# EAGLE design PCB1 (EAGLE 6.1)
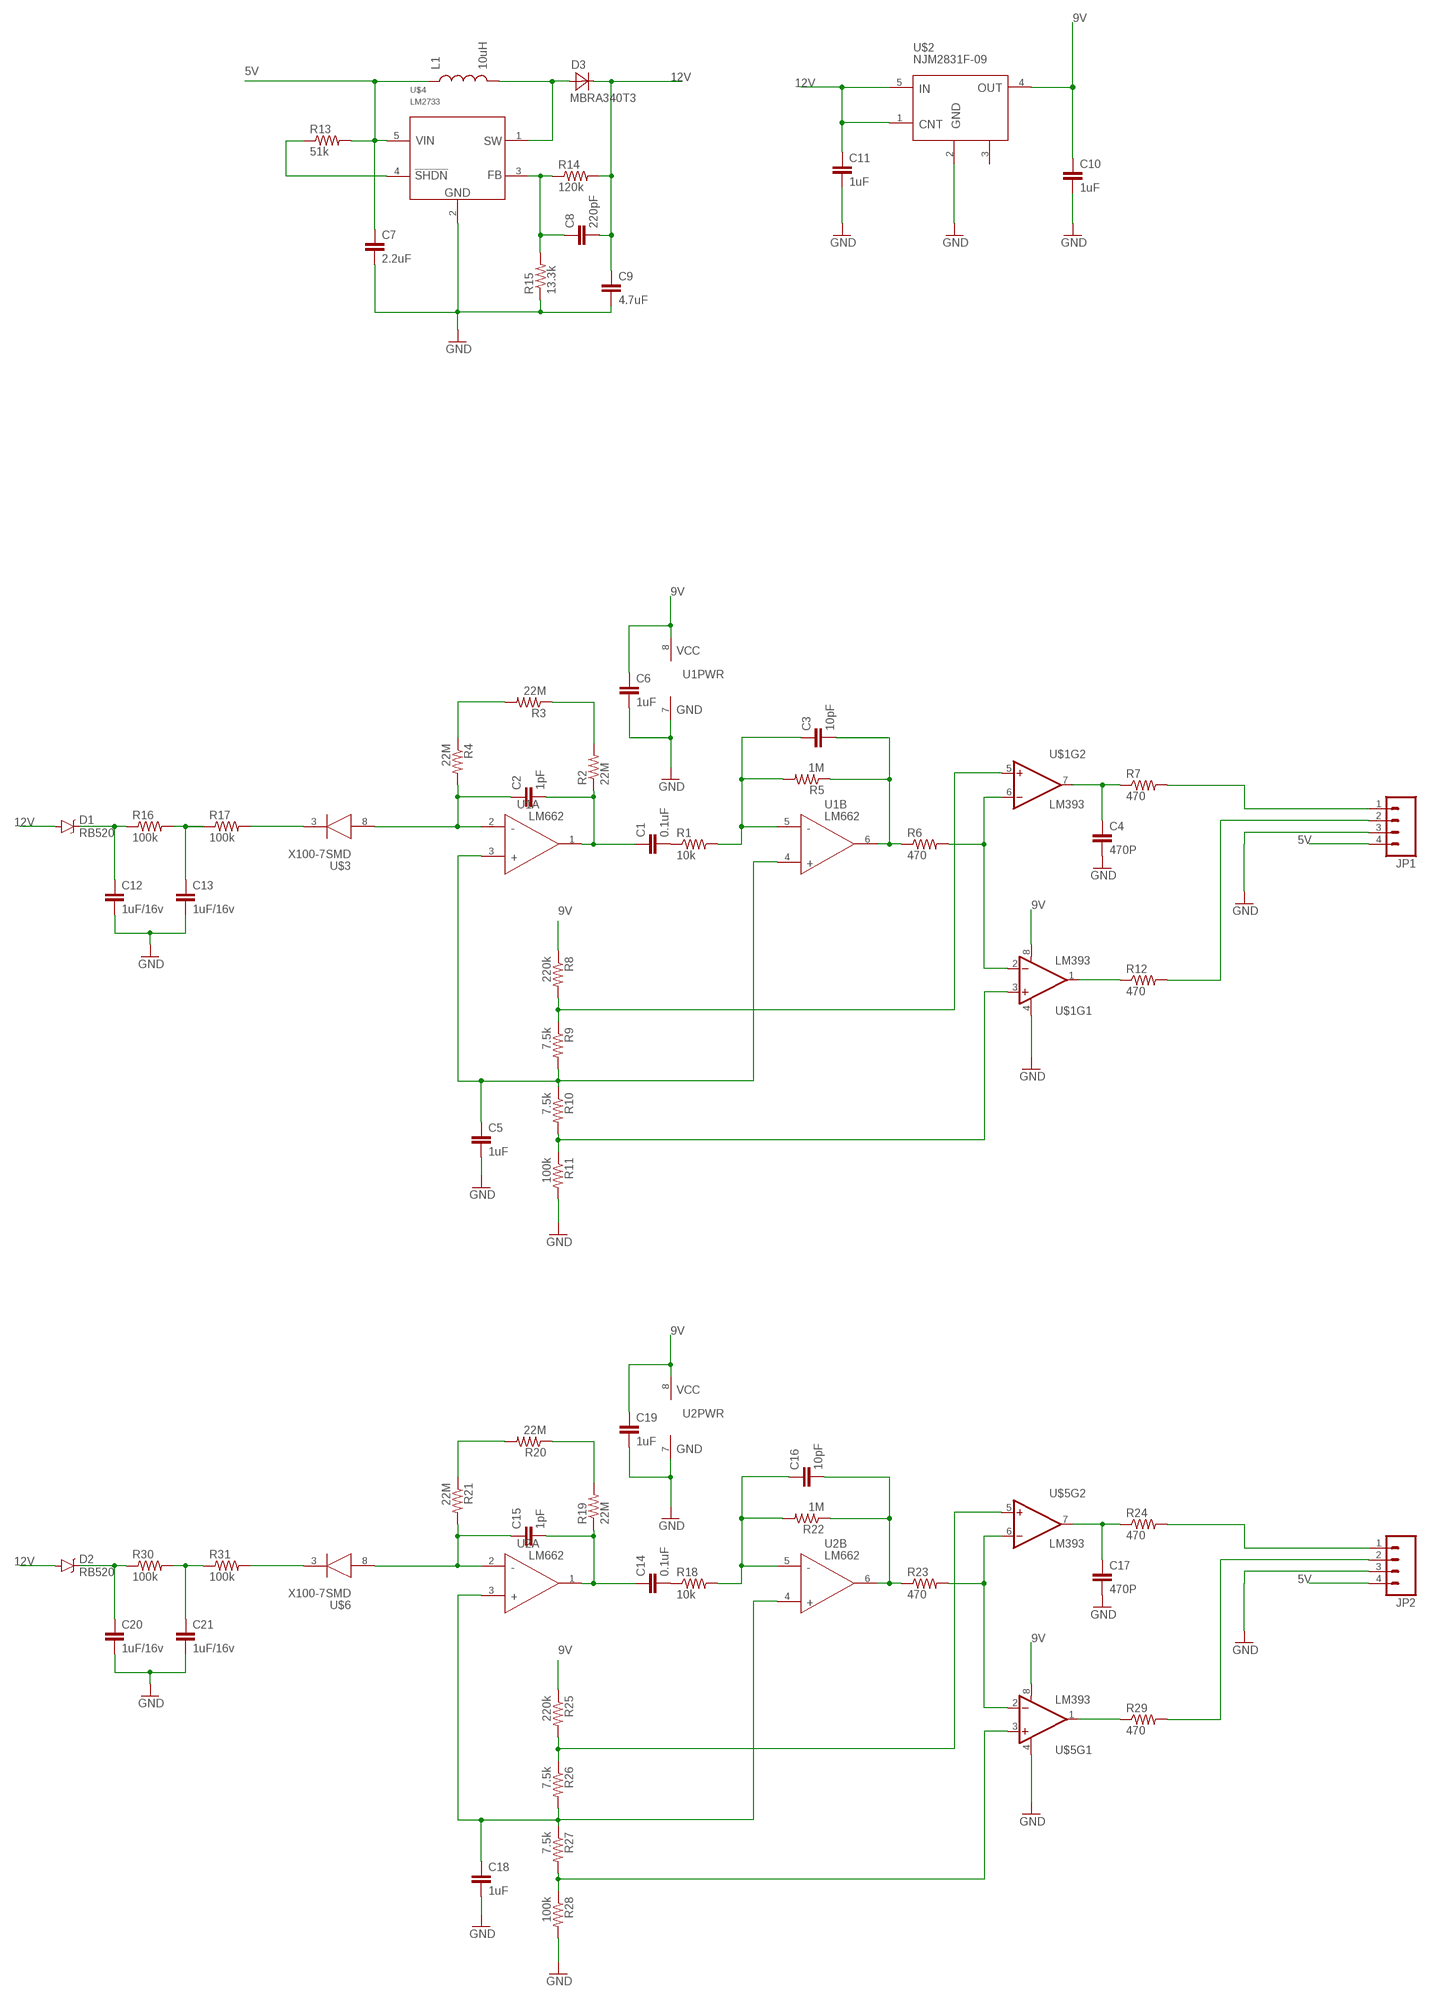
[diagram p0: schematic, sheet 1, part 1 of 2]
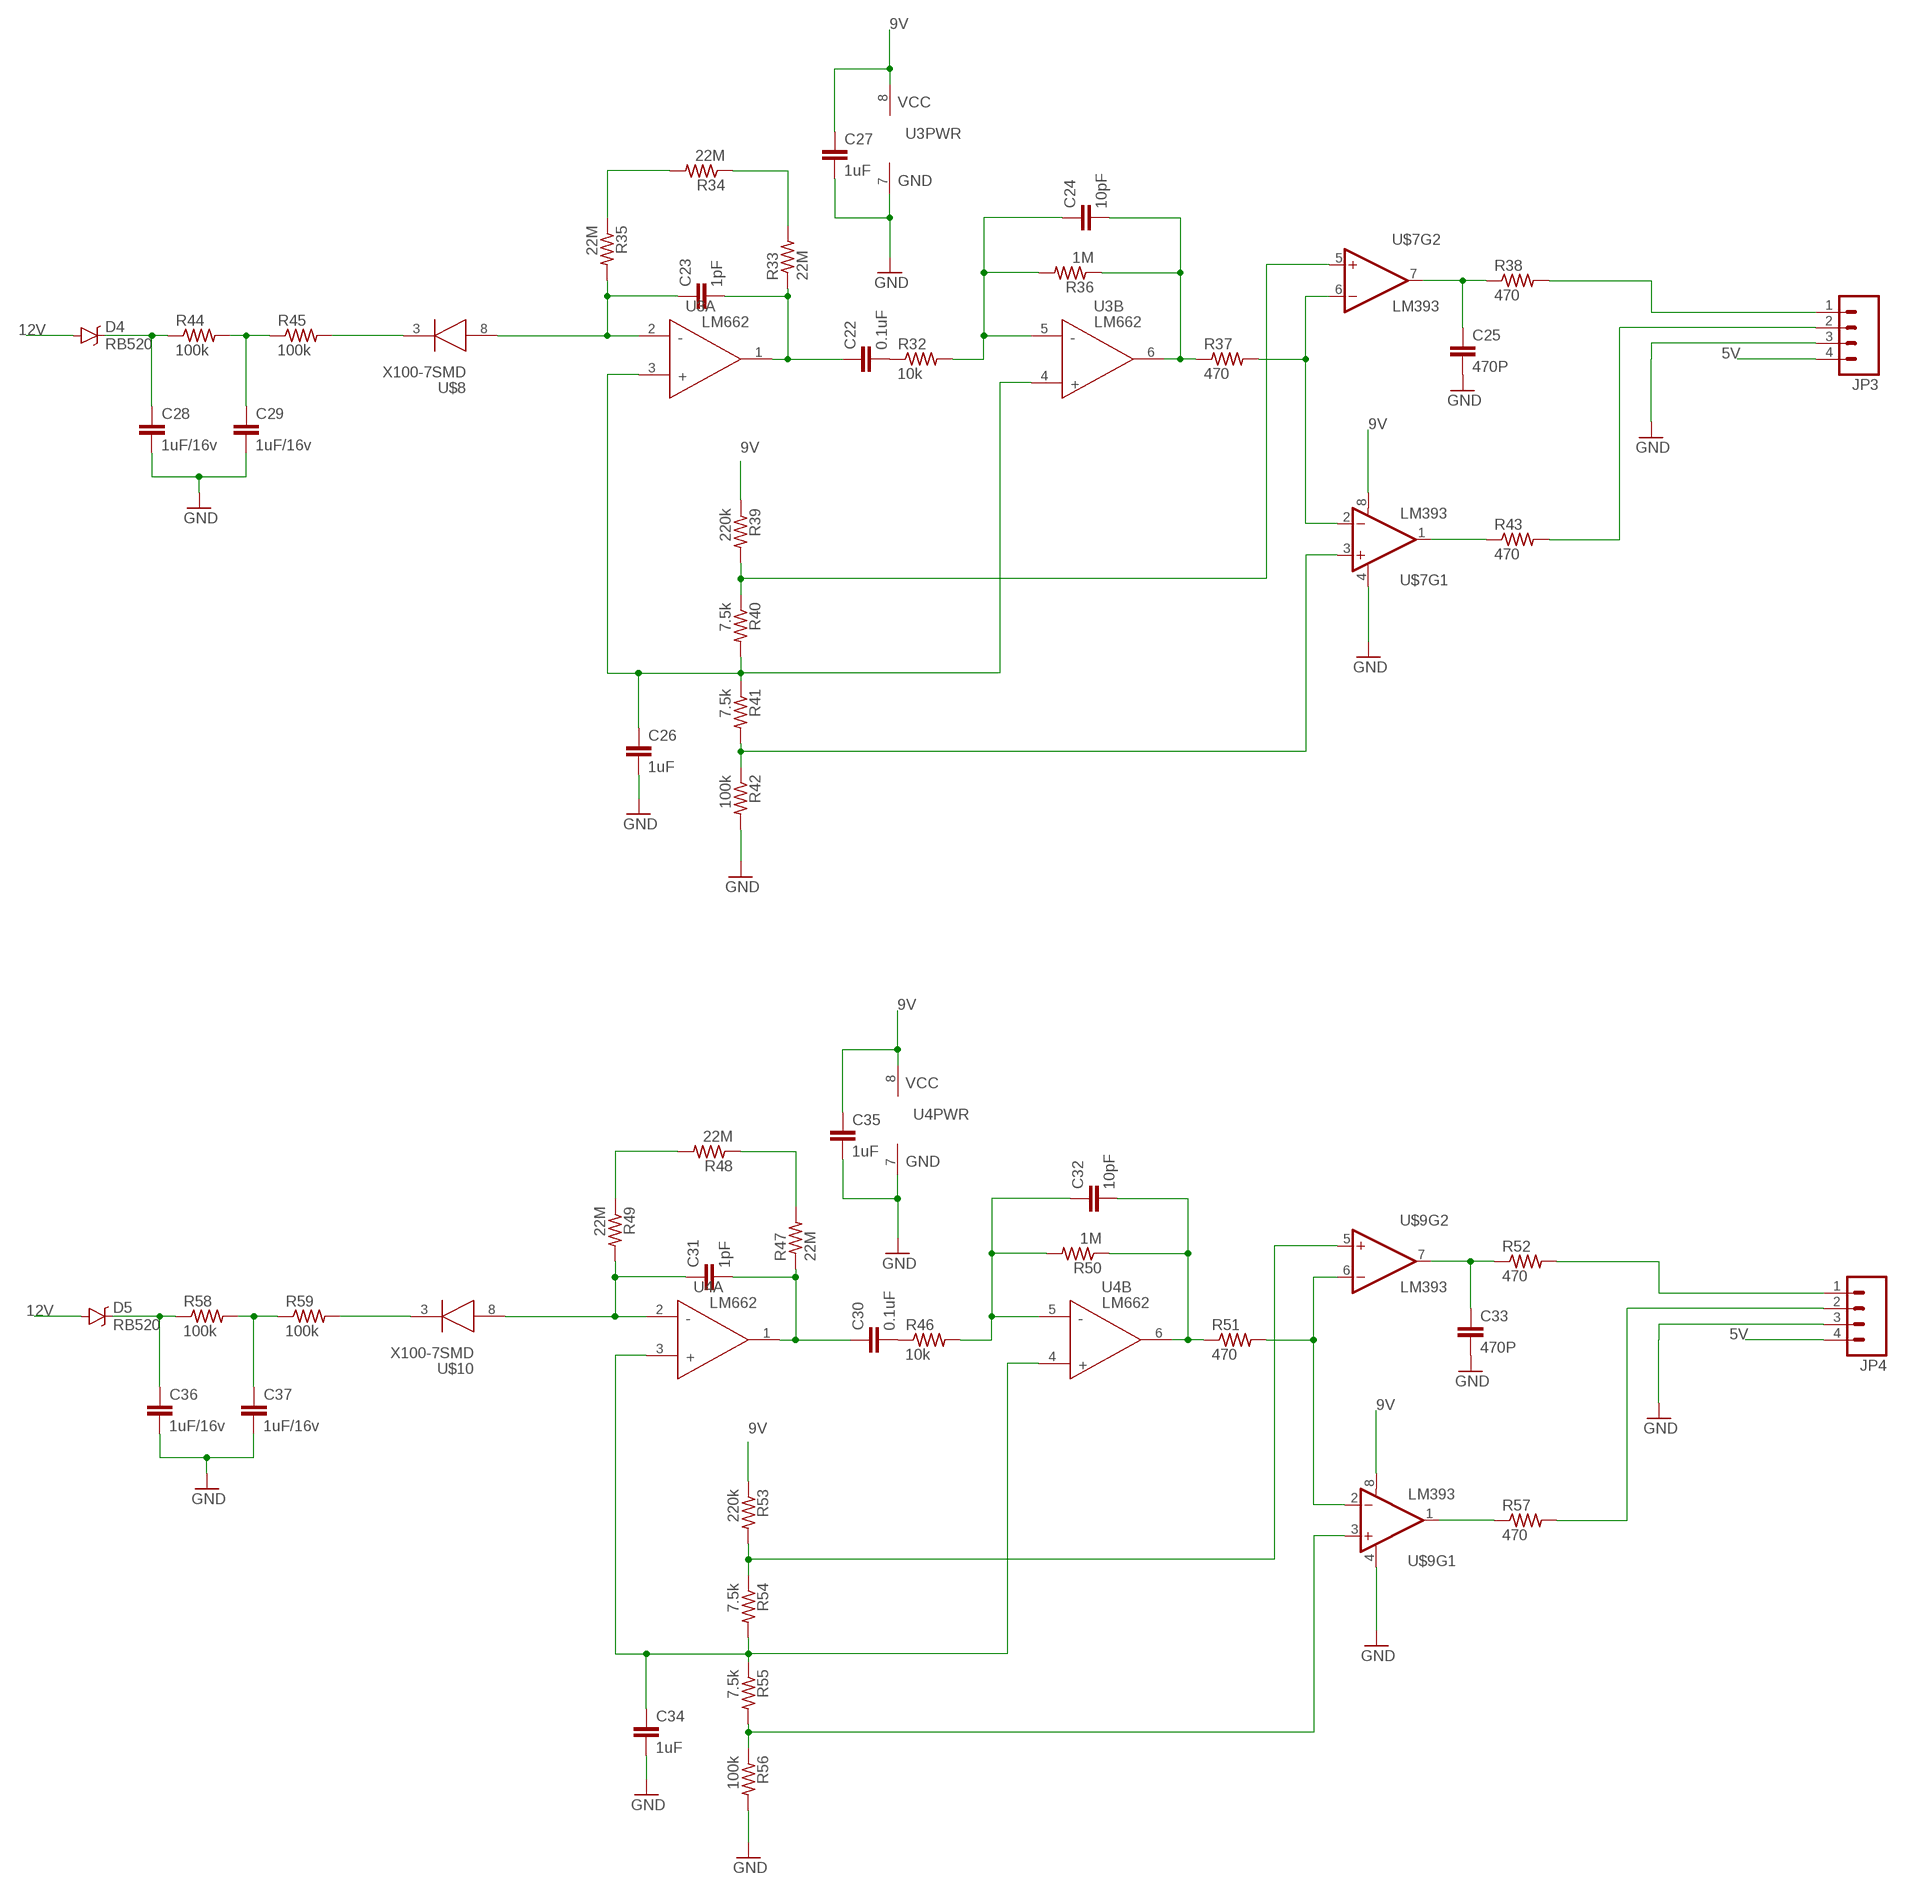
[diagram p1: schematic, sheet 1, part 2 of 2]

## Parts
C1  0.1uF  C-EUC1206  [C1206]
C2  1pF  C-EUC1206  [C1206]
C3  10pF  C-EUC1206  [C1206]
C4  470P  C-EUC1206  [C1206]
C5  1uF  C-EUC1206  [C1206]
C6  1uF  C-EUC1206  [C1206]
C7  2.2uF  C-EUC1206  [C1206]
C8  220pF  C-EUC1206  [C1206]
C9  4.7uF  C-EUC1206  [C1206]
C10  1uF  C-EUC1206  [C1206]
C11  1uF  C-EUC1206  [C1206]
C12  1uF/16v  C-EUC1206  [C1206]
C13  1uF/16v  C-EUC1206  [C1206]
C14  0.1uF  C-EUC1206  [C1206]
C15  1pF  C-EUC1206  [C1206]
C16  10pF  CAP0603-CAP  [0603-CAP]
C17  470P  C-EUC1206  [C1206]
C18  1uF  C-EUC1206  [C1206]
C19  1uF  C-EUC1206  [C1206]
C20  1uF/16v  C-EUC1206  [C1206]
C21  1uF/16v  C-EUC1206  [C1206]
C22  0.1uF  C-EUC1206  [C1206]
C23  1pF  C-EUC1206  [C1206]
C24  10pF  C-EUC1206  [C1206]
C25  470P  C-EUC1206  [C1206]
C26  1uF  C-EUC1206  [C1206]
C27  1uF  C-EUC1206  [C1206]
C28  1uF/16v  C-EUC1206  [C1206]
C29  1uF/16v  C-EUC1206  [C1206]
C30  0.1uF  C-EUC1206  [C1206]
C31  1pF  C-EUC1206  [C1206]
C32  10pF  C-EUC1206  [C1206]
C33  470P  C-EUC1206  [C1206]
C34  1uF  C-EUC1206  [C1206]
C35  1uF  C-EUC1206  [C1206]
C36  1uF/16v  C-EUC1206  [C1206]
C37  1uF/16v  C-EUC1206  [C1206]
D1  RB520  DIODE-SCHOTTKY-RB751  [SOD-523]
D2  RB520  DIODE-SCHOTTKY-RB751  [SOD-523]
D3  MBRA340T3  [SMA]
D4  RB520  DIODE-SCHOTTKY-RB751  [SOD-523]
D5  RB520  DIODE-SCHOTTKY-RB751  [SOD-523]
JP1  M04PTH  [1X04]
JP2  M04PTH  [1X04]
JP3  M04PTH  [1X04]
JP4  M04PTH  [1X04]
L1  10uH  INDUCTORBOURNS_SRN6045  [SRN6045]
R1  10k  R-US_R1206  [R1206]
R2  22M  R-US_R1206  [R1206]
R3  22M  R-US_R1206  [R1206]
R4  22M  R-US_R1206  [R1206]
R5  1M  R-US_R1206  [R1206]
R6  470  R-US_R1206  [R1206]
R7  470  R-US_R1206  [R1206]
R8  220k  R-US_R1206  [R1206]
R9  7.5k  R-US_R1206  [R1206]
R10  7.5k  R-US_R1206  [R1206]
R11  100k  R-US_R1206  [R1206]
R12  470  R-US_R1206  [R1206]
R13  51k  R-US_R1206  [R1206]
R14  120k  R-US_R1206  [R1206]
R15  13.3k  R-US_R1206  [R1206]
R16  100k  R-US_R1206  [R1206]
R17  100k  R-US_R1206  [R1206]
R18  10k  R-US_R1206  [R1206]
R19  22M  R-US_R1206  [R1206]
R20  22M  R-US_R1206  [R1206]
R21  22M  R-US_R1206  [R1206]
R22  1M  R-US_R1206  [R1206]
R23  470  R-US_R1206  [R1206]
R24  470  R-US_R1206  [R1206]
R25  220k  R-US_R1206  [R1206]
R26  7.5k  R-US_R1206  [R1206]
R27  7.5k  R-US_R1206  [R1206]
R28  100k  R-US_R1206  [R1206]
R29  470  R-US_R1206  [R1206]
R30  100k  R-US_R1206  [R1206]
R31  100k  R-US_R1206  [R1206]
R32  10k  R-US_R1206  [R1206]
R33  22M  R-US_R1206  [R1206]
R34  22M  R-US_R1206  [R1206]
R35  22M  R-US_R1206  [R1206]
R36  1M  R-US_R1206  [R1206]
R37  470  R-US_R1206  [R1206]
R38  470  R-US_R1206  [R1206]
R39  220k  R-US_R1206  [R1206]
R40  7.5k  R-US_R1206  [R1206]
R41  7.5k  R-US_R1206  [R1206]
R42  100k  R-US_R1206  [R1206]
R43  470  R-US_R1206  [R1206]
R44  100k  R-US_R1206  [R1206]
R45  100k  R-US_R1206  [R1206]
R46  10k  R-US_R1206  [R1206]
R47  22M  R-US_R1206  [R1206]
R48  22M  R-US_R1206  [R1206]
R49  22M  R-US_R1206  [R1206]
R50  1M  R-US_R1206  [R1206]
R51  470  R-US_R1206  [R1206]
R52  470  R-US_R1206  [R1206]
R53  220k  R-US_R1206  [R1206]
R54  7.5k  R-US_R1206  [R1206]
R55  7.5k  R-US_R1206  [R1206]
R56  100k  R-US_R1206  [R1206]
R57  470  R-US_R1206  [R1206]
R58  100k  R-US_R1206  [R1206]
R59  100k  R-US_R1206  [R1206]
U1  LM662  [SO08]
U2  LM662  [SO08]
U3  LM662  [SO08]
U4  LM662  [SO08]
U$1  LM393  [SO08]
U$2  NJM2831F-09  [SOT23-5]
U$3  X100-7SMD  [X100-7SMD]
U$4  LM2733  [SOT23-5]
U$5  LM393  [SO08]
U$6  X100-7SMD  [X100-7SMD]
U$7  LM393  [SO08]
U$8  X100-7SMD  [X100-7SMD]
U$9  LM393  [SO08]
U$10  X100-7SMD  [X100-7SMD]

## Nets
5V: C7.1 JP1.4 JP2.4 JP3.4 JP4.4 L1.1 R13.2 U$4.5
9V: C6.1 C10.1 C19.1 C27.1 C35.1 R8.1 R25.1 R39.1 R53.1 U1.8 U2.8 U3.8 U4.8 U$1.8(V+) U$2.4 U$5.8(V+) U$7.8(V+) U$9.8(V+)
12V: C8.2 C9.1 C11.1 D1.A D2.A D3.C D4.A D5.A R14.2 U$2.1 U$2.5
GND: C4.2 C5.2 C6.2 C7.2 C9.2 C10.2 C11.2 C12.2 C13.2 C17.2 C18.2 C19.2 C20.2 C21.2 C25.2 C26.2 C27.2 C28.2 C29.2 C33.2 C34.2 C35.2 C36.2 C37.2 JP1.3 JP2.3 JP3.3 JP4.3 R11.2 R15.1 R28.2 R42.2 R56.2 U1.7 U2.7 U3.7 U4.7 U$1.4(V-) U$2.2 U$4.2 U$5.4(V-) U$7.4(V-) U$9.4(V-)
N$1: C1.1 C2.2 R2.1 U1.1
N$2: C1.2 R1.1
N$3: C3.1 R1.2 R5.2 U1.5
N$4: R2.2 R3.1
N$5: R3.2 R4.1
N$6: C2.1 R4.2 U1.2 U$3.8
N$7: C3.2 R5.1 R6.1 U1.6
N$8: R6.2 U$1.2(-IN) U$1.6(-IN)
N$9: C4.1 R7.1 U$1.7(OUT)
N$10: R8.2 R9.1 U$1.5(+IN)
N$11: C5.1 R9.2 R10.1 U1.3 U1.4
N$12: R10.2 R11.1 U$1.3(+IN)
N$13: C12.1 D1.C R16.1
N$14: D3.A L1.2 U$4.1
N$15: C13.1 R16.2 R17.1
N$16: R12.1 U$1.1(OUT)
N$17: JP1.2 R12.2
N$18: R13.1 U$4.4
N$19: JP1.1 R7.2
N$20: R17.2 U$3.3
N$21: C8.1 R14.1 R15.2 U$4.3
N$22: C14.1 C15.2 R19.1 U2.1
N$23: C14.2 R18.1
N$24: C16.1 R18.2 R22.2 U2.5
N$25: R19.2 R20.1
N$26: R20.2 R21.1
N$27: C15.1 R21.2 U2.2 U$6.8
N$28: C16.2 R22.1 R23.1 U2.6
N$29: R23.2 U$5.2(-IN) U$5.6(-IN)
N$30: C17.1 R24.1 U$5.7(OUT)
N$31: R25.2 R26.1 U$5.5(+IN)
N$32: C18.1 R26.2 R27.1 U2.3 U2.4
N$33: R27.2 R28.1 U$5.3(+IN)
N$34: R29.1 U$5.1(OUT)
N$35: JP2.2 R29.2
N$36: JP2.1 R24.2
N$37: C20.1 D2.C R30.1
N$38: C21.1 R30.2 R31.1
N$39: R31.2 U$6.3
N$40: C22.1 C23.2 R33.1 U3.1
N$41: C22.2 R32.1
N$42: C24.1 R32.2 R36.2 U3.5
N$43: R33.2 R34.1
N$44: R34.2 R35.1
N$45: C23.1 R35.2 U3.2 U$8.8
N$46: C24.2 R36.1 R37.1 U3.6
N$47: R37.2 U$7.2(-IN) U$7.6(-IN)
N$48: C25.1 R38.1 U$7.7(OUT)
N$49: R39.2 R40.1 U$7.5(+IN)
N$50: C26.1 R40.2 R41.1 U3.3 U3.4
N$51: R41.2 R42.1 U$7.3(+IN)
N$52: R43.1 U$7.1(OUT)
N$53: JP3.2 R43.2
N$54: JP3.1 R38.2
N$55: C28.1 D4.C R44.1
N$56: C29.1 R44.2 R45.1
N$57: R45.2 U$8.3
N$58: C30.1 C31.2 R47.1 U4.1
N$59: C30.2 R46.1
N$60: C32.1 R46.2 R50.2 U4.5
N$61: R47.2 R48.1
N$62: R48.2 R49.1
N$63: C31.1 R49.2 U4.2 U$10.8
N$64: C32.2 R50.1 R51.1 U4.6
N$65: R51.2 U$9.2(-IN) U$9.6(-IN)
N$66: C33.1 R52.1 U$9.7(OUT)
N$67: R53.2 R54.1 U$9.5(+IN)
N$68: C34.1 R54.2 R55.1 U4.3 U4.4
N$69: R55.2 R56.1 U$9.3(+IN)
N$70: R57.1 U$9.1(OUT)
N$71: JP4.2 R57.2
N$72: JP4.1 R52.2
N$73: C36.1 D5.C R58.1
N$74: C37.1 R58.2 R59.1
N$75: R59.2 U$10.3
Unconnected: U$2.3

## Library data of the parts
C1-C15 C17-C37 = resistor:C-EU: CAPACITOR, European symbol
C16 = SparkFun-Capacitors:CAP: Capacitor
D1 D2 D4 D5 = SparkFun-DiscreteSemi:DIODE-SCHOTTKY: Schottky diodes in SFE's production catalog; PROD_ID: DIO-11018; VALUE: RB751
D3 = diode:MBRA340T3: Surface Mount Schottky Power Rectifier
JP1-JP4 = SparkFun-Connectors:M04: Header 4 Standard 4-pin 0.1" header. Use with straight break away headers (SKU : PRT-00116), right angle break away headers (PRT-00553), swiss pins (PRT-00743), machine pins (PRT-00117), and female headers (PRT-00115). Molex polarized connector foot print use with SKU : PRT-08231 with associated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
L1 = SparkFun-Passives:INDUCTOR: Inductors; PROD_ID: NDUC-11627; VALUE: 33uH
R1-R59 = resistor:R-US_: RESISTOR, American symbol
U1-U4 = LMC662:LM662
U$1 U$5 U$7 U$9 = SparkFun-AnalogIC:LM393: Low-voltage comparator
U$2 = NJM2831F-09:NJM2831F-09
U$3 U$6 U$8 U$10 = X100-7SMD:X100-7SMD
U$4 = LM2733:LM2733

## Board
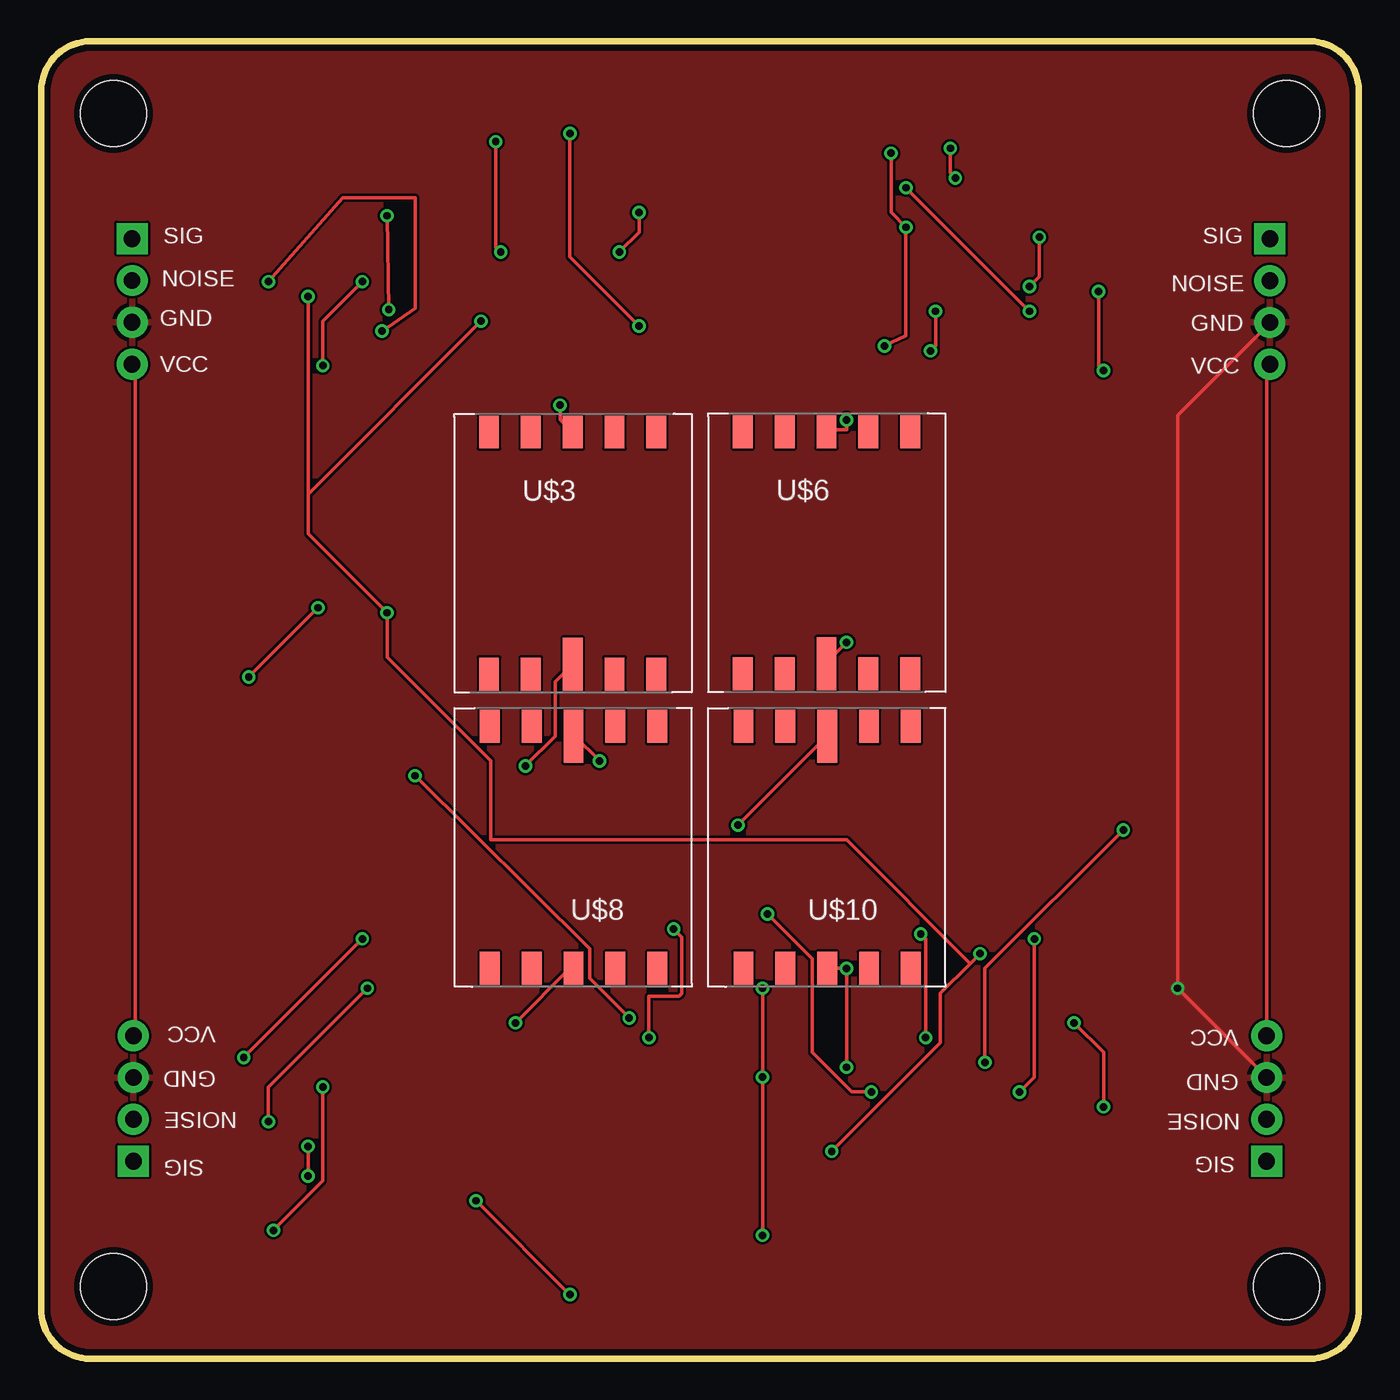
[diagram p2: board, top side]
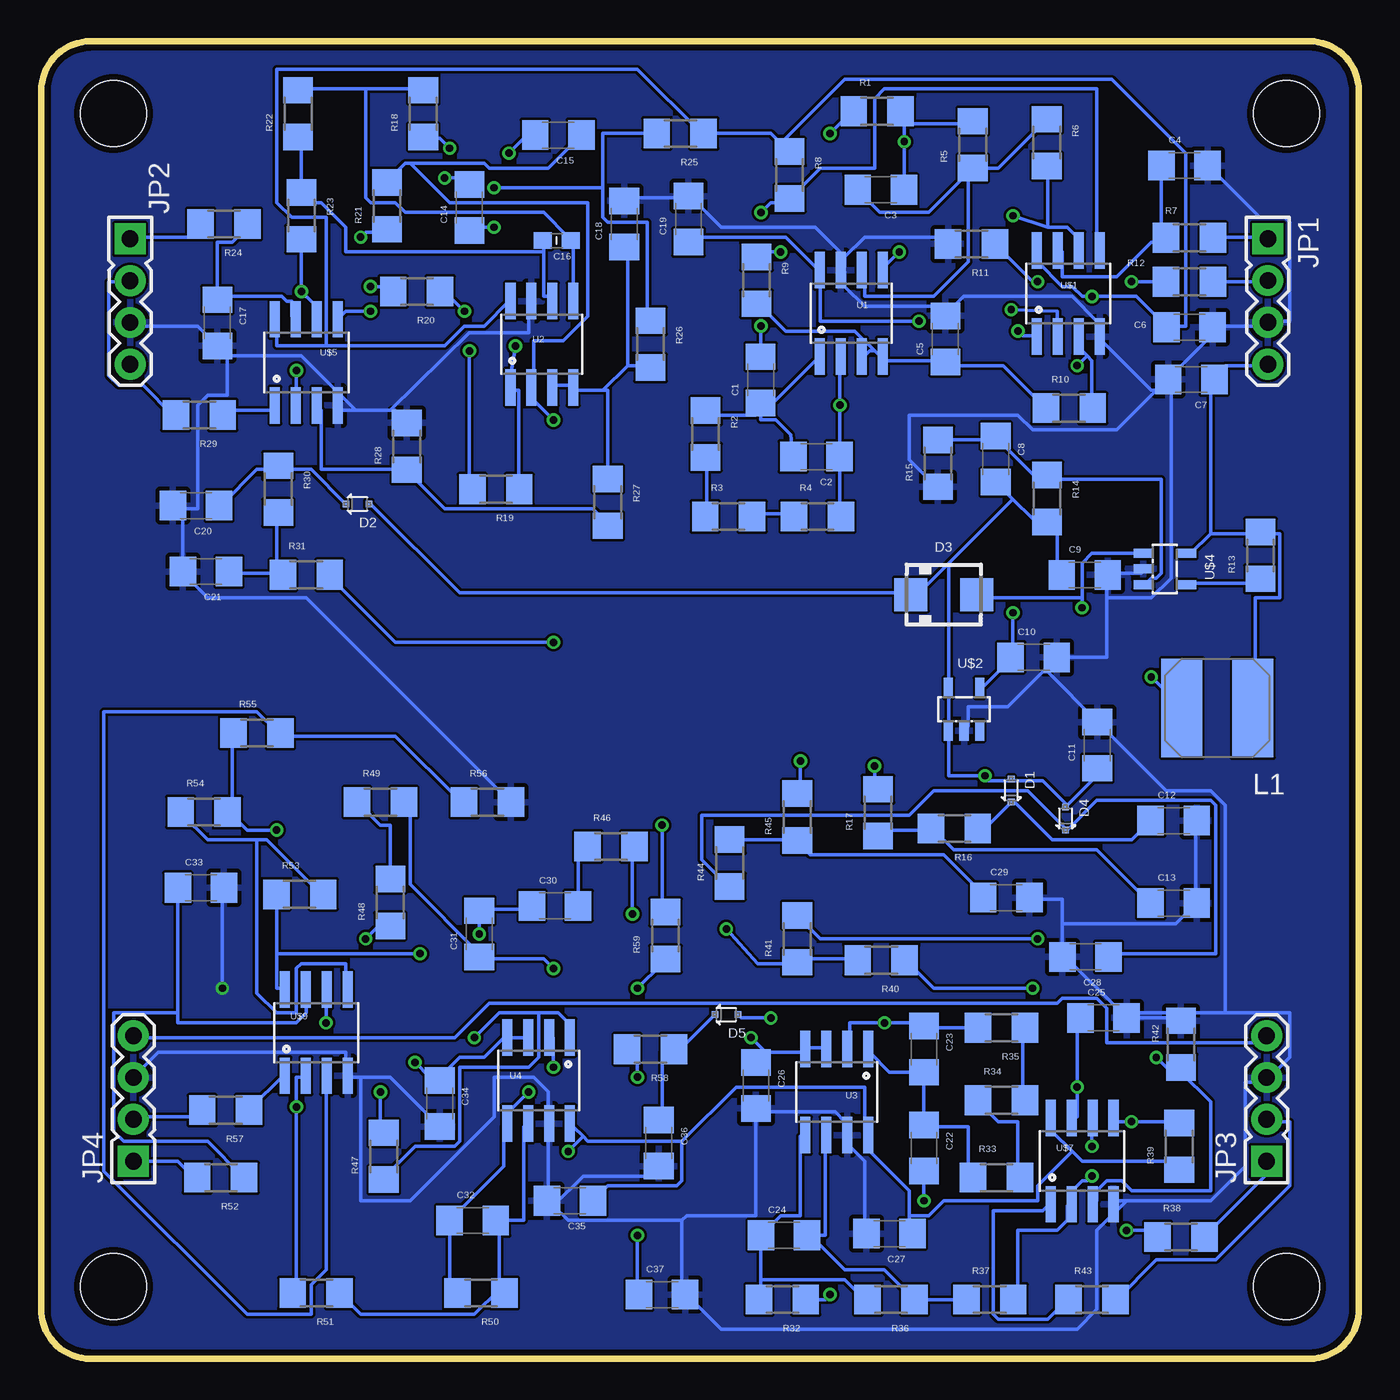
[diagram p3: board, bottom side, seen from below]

Size 80 x 80 mm. Coordinates in mm from the lower left corner, seen from the top.
Outline: 3,0 77,0
Outline: 0,77 0,2.8
Outline: 77,0 3,0
Outline: 0,2.8 0,77
Outline: 0,77 arc-90 3,80 77,80 arc-90 80,77 80,2.8 arc-86 77,0
Outline: 3,0 arc-86 0,2.8
Copper layers (1*16): Top 0.0356mm / dielectric 1.5011mm / Bottom 0.0356mm
Design rules: minimum track width 6mil, minimum drill 13mil, track to track 6mil, track to pad 6mil, pad to pad 6mil, via to via 6mil, smd to smd 6mil, copper to edge 15mil, drill to drill 6mil, minimum pad ring 7mil, minimum via ring 7mil, stop-mask expansion 3mil, vias tented up to drill 0mil, thermal gap 10mil
Holes 4 mm at 75.6,4.4 4.4,4.4 4.4,75.6 75.6,75.6

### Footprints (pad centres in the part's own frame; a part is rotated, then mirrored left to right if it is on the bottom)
C1206 = smd 1.6 x 1.8: 1 -1.4,0; 2 1.4,0
0603-CAP = smd 1.1 x 1: 1 -0.85,0; 2 0.85,0
SOD-523 = smd 0.4 x 0.4: A -0.7,0; C 0.7,0
SMA = smd 2 x 2: A 2,0; C -2,0
1X04 = drill 1.016 pad 1.88 square: 1 0,0 | drill 1.016 pad 1.88: 2 2.54,0; 3 5.08,0; 4 7.62,0
SRN6045 = smd 2.5 x 6: 1 -2.175,-0.175; 2 2.125,-0.175
R1206 = smd 1.6 x 1.803: 1 -1.422,0; 2 1.422,0
SO08 = smd 0.61 x 2.21: 1 -1.905,-2.616; 2 -0.635,-2.616; 3 0.635,-2.616; 4 1.905,-2.616; 5 1.905,2.616; 6 0.635,2.616; 7 -0.635,2.616; 8 -1.905,2.616
SOT23-5 = smd 0.55 x 1.2: 1 -0.95,-1.3; 2 0,-1.3; 3 0.95,-1.3; 4 0.95,1.3; 5 -0.95,1.3
X100-7SMD = smd 1.2 x 2: 1 0,0; 2 2.54,0; 4 7.62,0; 5 10.16,0; 6 10.16,14.7; 7 7.62,14.7; 8 5.08,14.7; 9 2.54,14.7; 10 0,14.7 | smd 1.2 x 3.2: 3 5.08,0.6

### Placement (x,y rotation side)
C1  36.32,59.44 90 bottom
C2  32.93,54.78 180 bottom
C3  29.02,70.98 180 bottom
C4  10.58,72.45 0 bottom
C5  25.1,61.92 90 bottom
C6  10.28,62.63 0 bottom
C7  10.17,59.46 180 bottom
C8  22.04,54.63 270 bottom
C9  16.64,47.59 0 bottom
C10  19.74,42.59 0 bottom
C11  15.88,37.26 90 bottom
C12  11.24,32.68 0 bottom
C13  11.24,27.67 0 bottom
C14  54,69.9 90 bottom
C15  48.6,74.3 180 bottom
C16  48.7,67.9 180 bottom
C17  69.3,62.9 270 bottom
C18  44.6,68.9 90 bottom
C19  40.7,69.2 90 bottom
C20  70.6,51.8 180 bottom
C21  70,47.8 180 bottom
C22  26.4,12.8 270 bottom
C23  26.4,18.8 270 bottom
C24  34.9,7.5 0 bottom
C25  15.5,20.7 0 bottom
C26  36.6,16.6 270 bottom
C27  28.5,7.6 180 bottom
C28  16.6,24.4 180 bottom
C29  21.4,28 0 bottom
C30  48.8,27.5 0 bottom
C31  53.4,25.8 90 bottom
C32  53.8,8.4 0 bottom
C33  70.3,28.6 0 bottom
C34  55.8,15.5 270 bottom
C35  47.9,9.6 180 bottom
C36  42.5,13.1 270 bottom
C37  42.3,3.9 0 bottom
D1  21.1,34.5 270 bottom
D2  60.8,51.9 180 bottom
D3  25.2,46.4 0 bottom
D4  17.8,32.8 270 bottom
D5  38.4,20.9 180 bottom
JP1  5.52,68.01 270 bottom
JP2  74.6,68 270 bottom
JP3  5.6,12 90 bottom
JP4  74.4,12 90 bottom
L1  8.62,39.34 180 bottom
R1  29.24,75.74 0 bottom
R2  39.66,56.15 270 bottom
R3  38.26,51.14 0 bottom
R4  32.87,51.14 0 bottom
R5  23.44,73.72 90 bottom
R6  18.95,73.84 270 bottom
R7  10.28,68.06 0 bottom
R8  34.56,71.88 270 bottom
R9  36.57,65.48 270 bottom
R10  17.58,57.72 0 bottom
R11  23.52,67.69 180 bottom
R12  10.28,65.39 0 bottom
R13  5.97,48.78 90 bottom
R14  18.93,52.23 270 bottom
R15  25.55,54.37 90 bottom
R16  24.56,32.2 180 bottom
R17  29.19,33.16 90 bottom
R18  56.8,75.6 90 bottom
R19  52.4,52.8 180 bottom
R20  57.2,64.8 180 bottom
R21  59,70 90 bottom
R22  64.4,75.6 90 bottom
R23  64.2,69.4 270 bottom
R24  68.9,68.9 180 bottom
R25  41.2,74.4 180 bottom
R26  43,61.6 270 bottom
R27  45.6,52 270 bottom
R28  57.8,55.4 90 bottom
R29  70.4,57.3 180 bottom
R30  65.6,52.8 270 bottom
R31  63.9,47.6 0 bottom
R32  35,3.6 180 bottom
R33  22,11 0 bottom
R34  21.7,15.7 0 bottom
R35  21.7,20.1 180 bottom
R36  28.4,3.6 180 bottom
R37  22.4,3.6 0 bottom
R38  10.8,7.4 0 bottom
R39  10.9,12.9 90 bottom
R40  29,24.2 180 bottom
R41  34.1,25.5 90 bottom
R42  10.8,19.1 90 bottom
R43  16.2,3.6 0 bottom
R44  38.2,30.1 90 bottom
R45  34.1,32.9 90 bottom
R46  45.4,31.1 0 bottom
R47  59.2,12.3 90 bottom
R48  58.8,27.7 90 bottom
R49  59.4,33.8 0 bottom
R50  53.3,4 180 bottom
R51  63.3,4 180 bottom
R52  69.1,11 180 bottom
R53  64.3,28.2 0 bottom
R54  70.1,33.2 0 bottom
R55  66.9,38 0 bottom
R56  52.9,33.8 0 bottom
R57  68.8,15.1 180 bottom
R58  43,18.8 180 bottom
R59  42.1,25.7 90 bottom
U1  30.82,63.48 0 bottom
U2  49.6,61.6 0 bottom
U3  31.7,16.2 180 bottom
U4  49.8,16.9 180 bottom
U$1  17.64,64.68 0 bottom
U$2  23.97,39.44 0 bottom
U$3  27.19,41.57 0 top
U$4  11.78,47.96 270 bottom
U$5  63.9,60.5 0 bottom
U$6  42.6,41.6 0 top
U$7  16.8,12 0 bottom
U$8  37.4,38.4 180 top
U$9  63.3,19.8 0 bottom
U$10  52.8,38.4 180 top

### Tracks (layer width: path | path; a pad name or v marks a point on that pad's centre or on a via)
5V
  Top 0.2: JP4.4 74.4,19.8 74.4,60.3 JP2.4 | JP3.4 5.7,19.8 5.7,60.3 JP1.4
  Bottom 0.2: 9,50.1 10.2,48.9 U$4.5 | 9,50.1 6,50.1 R13.2 5.7,50.1 4.8,50.1 4.8,46.2 6.3,46.2 6.3,39.6 L1.1 | JP1.4 5.7,60.3 8.1,60.3 8.7,59.7 C7.1 9,59.4 9,50.1 | JP4.4 74.4,19.5 54.9,19.5 52.8,21.6 18.3,21.6 18,21.9 15.9,21.9 15.3,21.3 15.3,19.2 6,19.2 5.7,19.5 JP3.4
9V  (via drill 0.45)
  Top 0.2: 56.4,24 54.6,22.2 54.6,19.2 v48,12.6 | 56.4,24 v57,24.6 | v16.2,64.5 16.2,52.5 | 16.2,52.5 16.2,50.1 v21,45.3 21,42.6 27.3,36.3 27.3,31.5 48.9,31.5 56.4,24 | 16.2,52.5 v26.7,63
  Bottom 0.2: 17.4,12.6 18.6,13.8 18.6,14.4 U$7.8 | 17.4,12.6 16.8,12 11.4,12 11.1,11.7 R39.1 | 27.3,8.7 27.3,10.2 29.7,12.6 29.7,13.5 U3.8 30,13.8 30,16.5 37.8,16.5 41.1,13.2 | 27.3,8.7 27.3,7.8 C27.1 | 65.7,24.6 65.7,22.5 65.4,22.5 U$9.8 | 65.7,24.6 65.7,28.2 R53.1 | C35.1 45.6,10.5 41.4,10.5 41.1,10.8 41.1,13.2 | 41.1,13.2 46.8,13.2 47.1,13.5 | 47.1,13.5 47.7,14.1 U4.8 | v57,24.6 65.7,24.6 | 47.1,13.5 v48,12.6 | 17.4,12.6 19.5,10.5 19.5,9.6 25.2,9.6 26.1,8.7 27.3,8.7 | 62.7,61.5 55.5,61.5 54.3,62.7 53.1,62.7 51.6,64.2 U2.8 | 62.7,61.5 65.7,61.5 65.7,63 U$5.8 | C19.1 40.5,67.8 40.2,68.1 34.8,68.1 33,66.3 U1.8 32.7,66 32.7,63 v26.7,63 | 35.1,73.8 35.7,74.4 39.6,74.4 R25.1 39.9,74.4 43.8,78.3 65.7,78.3 65.7,70.2 64.8,69.3 62.7,69.3 62.7,61.5 | 35.1,73.8 34.8,73.5 R8.1 35.1,73.8 | U$2.4 22.8,40.8 21.3,42.3 C10.1 21,42.6 v21,45.3 | U$1.8 19.5,67.2 19.5,66.6 18,65.1 17.4,65.1 16.8,64.5 v16.2,64.5 13.5,64.5 11.7,62.7 C6.1 11.4,62.7 10.5,62.7 10.5,73.2 15,77.7 31.2,77.7 35.1,73.8
12V  (via drill 0.45)
  Top 0.2: v35.7,20.7 33.3,23.1 33.3,24.9 v22.7,35.4
  Bottom 0.2: 17.7,33.6 15.6,35.7 C11.1 | 17.7,33.6 D4.A 17.7,33.6 | D5.A 37.5,20.7 v35.7,20.7 | D5.A 37.8,21 D5.A | 21,35.1 22.5,35.1 v22.7,35.4 24.9,35.4 24.9,38.1 U$2.1 24.9,38.4 24.9,40.5 U$2.5 24.9,40.8 24.9,48.3 | 21,35.1 D1.A 21,35.1 | 17.7,33.6 19.2,35.1 21,35.1 | C9.1 18.3,47.7 18.3,50.7 18.9,50.7 R14.2 19.2,51 19.8,51 21,52.2 | 21,52.2 21.9,53.1 C8.2 | D2.A 60,51.9 54.6,46.5 27.3,46.5 D3.C 27,46.5 26.7,46.5 24.9,48.3 | 24.9,48.3 21,52.2
GND  (via drill 0.45)
  Top 0.2: JP4.3 74.4,17.1 v69,22.5 69,57.3 74.4,62.7 JP2.3
  Bottom 0.2: C18.2 44.4,70.5 40.8,70.5 C19.2 40.5,70.5 38.7,68.7 33,68.7 31.2,66.9 | U1.7 31.2,66 31.2,65.1 30,63.9 25.5,63.9 25.2,63.6 C5.2 24.9,63.6 24,64.5 17.4,64.5 15.9,63 15.9,62.1 U$1.4 15.6,61.8 12.6,58.8 12.3,58.8 | 31.2,66.9 30,68.1 25.5,68.1 25.2,67.8 R11.2 | 31.2,66.9 31.2,66.3 U1.7 | 31.2,66.9 U1.7 | U$4.2 13.2,47.7 15,47.7 C9.2 15.3,47.4 15.3,46.2 | 19.2,41.7 18.6,42.3 C10.2 18.3,42.6 15.3,42.6 15.3,46.2 | 19.2,41.7 21.3,39.6 23.7,39.6 23.7,38.4 U$2.2 | 19.2,41.7 18.9,41.7 15.9,38.7 C11.2 15.6,38.4 11.7,34.5 9,34.5 8.1,33.6 8.1,21 | C4.2 9,72.3 6,69.3 4.5,69.3 4.2,69 4.2,63 5.4,63 JP1.3 5.7,62.7 8.7,62.7 C6.2 8.7,62.4 11.4,59.7 C7.2 | 12.3,58.8 11.7,59.4 C7.2 | 12.3,58.8 14.7,56.4 19.8,56.4 20.7,57.3 27.3,57.3 27.3,54.6 25.8,53.1 R15.1 | 12.3,58.8 C7.2 | 15.3,46.2 12.6,46.2 11.4,47.4 11.4,59.4 C7.2 | C17.2 70.5,62.7 74.4,62.7 JP2.3 | 60.9,57.6 61.8,57.6 U$5.4 | 60.9,57.6 58.8,57.6 | 58.8,57.6 58.5,57.6 57.9,57 R28.2 | 58.8,57.6 54,62.3 50.4,62.3 50.4,64.2 U2.7 | 68.7,60.9 C17.2 | 68.7,60.9 64.2,60.9 60.9,57.6 | 71.4,51.6 71.4,48 C21.2 71.4,47.7 69.9,46.2 63.9,46.2 51.6,33.9 R56.2 | 71.4,51.6 72,51.6 C20.2 71.4,51.6 | 68.7,60.9 68.7,58.5 69.9,58.5 70.5,57.9 70.5,51.6 71.4,51.6 | 68.7,60.9 C17.2 | C34.2 58.8,17.1 60.6,17.1 | 60.6,17.1 61.2,17.1 U$9.4 61.5,17.4 61.5,18.6 72.9,18.6 74.4,17.1 JP4.3 | v69,22.5 69,28.5 C33.2 | C27.2 30,7.8 30,12 30.9,12.9 30.9,13.5 U3.7 31.2,13.8 31.2,14.4 31.8,15 36.6,15 | 36.6,15 C26.2 36.6,15 | 41.1,8.4 41.1,3.9 C37.2 40.8,3.9 38.7,1.8 17.1,1.8 15.9,3 15.9,7.8 14.1,9.6 | 41.1,8.4 48,8.4 48.9,9.3 | 49.2,9.6 48.9,9.3 | 49.2,9.6 C35.2 | 48.9,9.3 47.1,11.1 43.2,11.1 42.6,11.7 C36.2
  Bottom 0.2: 48.9,9.3 C35.2 | 49.2,9.6 49.2,14.1 U4.7 49.2,14.4 49.2,16.2 50.1,17.1 52.5,17.1 52.5,14.7 57.6,9.6 60.6,9.6 60.6,17.1 | 49.2,9.6 C35.2 | 36.6,15 36.6,8.7 40.8,8.7 41.1,8.4 | 14.1,9.6 9,9.6 6.9,11.7 6.9,16.8 5.7,16.8 JP3.3 5.4,17.1 4.2,18.3 4.2,21 8.1,21 | 14.1,9.6 14.7,9.6 U$7.4 | C12.2 9.9,32.4 9.9,27.9 C13.2 9.9,27.6 11.1,26.4 18,26.4 | C25.2 10.8,20.7 R42.2 | 18,26.4 18,27.9 19.8,27.9 C29.2 | 18,26.4 18,24.6 C28.2 18,24.3 17.7,24.3 14.4,21 | 14.4,21 C25.2 | 14.4,21 8.1,21 | 14.4,21 C25.2
  pour Top: 3,80 77,80 arc-90 80,77 80,3 arc-90 77,0 3,0 arc-90 0,3 0,77.1 arc-90 2.9,80
  pour Bottom: 3,80 77,80 arc-90 80,77 80,3 arc-90 77,0 3,0 arc-90 0,3 0,77.1 arc-90 2.9,80
N$1
  Bottom 0.2: C2.2 34.5,56.1 35.4,57 36.3,57 C1.1 | R2.1 39.6,57.3 36.6,57.3 C1.1 | U1.1 33,60.6 36.3,57.3 C1.1
N$2  (via drill 0.45)
  Top 0.2: v36.3,62.7 32.1,66.9 v32.1,74.4
  Bottom 0.2: v36.3,62.7 36.3,60.3 C1.2 | v32.1,74.4 30.9,75.6 R1.1
N$3  (via drill 0.45)
  Top 0.2: v27.9,67.2 27.6,67.5 v27.6,73.9
  Bottom 0.2: 27.6,75 27.6,75.6 R1.2 27.6,75 | 27.6,75 v27.6,73.9 27.6,71.1 C3.1 | 27.6,75 23.7,75 R5.2 | v27.9,67.2 28.8,66.3 U1.5
N$4
  Bottom 0.2: R3.1 39.6,51.3 39.6,54.6 R2.2
N$5
  Bottom 0.2: R4.1 34.5,51.3 36.6,51.3 R3.2
N$6  (via drill 0.45)
  Top 0.2: v31.5,57.9 31.5,57 32.1,56.4 U$3.8
  Bottom 0.2: U1.2 31.5,60.6 v31.5,57.9 31.5,56.1 C2.1 31.5,55.8 31.5,51.3 R4.2
N$7
  Bottom 0.2: 23.7,72 26.1,69.6 29.1,69.6 30.3,70.8 C3.2 | 23.7,72 R5.1 | R6.1 19.2,75 21.9,72.3 23.4,72.3 R5.1 | 23.7,72 23.7,66.6 25.8,64.5 30,64.5 30,66 U1.6 | 23.7,72 R5.1
N$8  (via drill 0.45)
  Top 0.2: v21,69.4 v21.1,63.7
  Bottom 0.2: 18.9,68.7 18.9,72.3 R6.2 | 18.9,68.7 17.7,68.7 17.1,68.1 17.1,67.5 U$1.6 | v21.1,63.7 18.3,63.6 18.3,62.1 U$1.2 | 18.9,68.7 v21,69.4
N$9
  Bottom 0.2: C4.1 12,72.3 12,68.1 R7.1 12,67.8 12.6,67.8 14.7,65.7 18,65.7 18,67.2 U$1.7
N$10  (via drill 0.45)
  Top 0.2: v35.1,67.2 36.3,68.4 v36.3,69.6
  Bottom 0.2: v35.1,67.2 36.3,67.2 R9.1 | v36.3,69.6 35.7,70.2 34.8,70.2 R8.2 34.5,70.5 32.7,72.3 29.4,72.3 29.4,76.5 28.8,77.1 15.9,77.1 15.9,67.5 U$1.5
N$11
  Bottom 0.2: R10.1 19.2,57.9 21.6,60.3 24.9,60.3 C5.1 25.2,60.6 28.8,60.6 U1.4 29.1,60.9 29.4,61.2 | 29.4,61.2 30.6,62.4 34.8,62.4 36.3,63.9 R9.2 | 29.4,61.2 29.7,61.2 30,60.9 U1.3
N$12  (via drill 0.45)
  Top 0.2: v19.5,65.4 17.1,63 v17.1,60.3
  Bottom 0.2: 16.5,60.9 16.8,61.2 16.8,61.8 U$1.3 | 16.5,60.9 16.2,60.6 16.2,57.9 R10.2 | v19.5,65.4 19.8,65.4 21.9,67.5 R11.1 | 16.5,60.9 v17.1,60.3
N$13
  Bottom 0.2: D1.C 22.5,32.4 23.1,32.4 R16.1 | D1.C 21,33.9 | 21,33.9 D1.C | 21,33.9 18.6,31.5 13.8,31.5 12.9,32.4 C12.1 | 21,33.9 D1.C
N$14  (via drill 0.45)
  Top 0.2: v12.6,41.4 v16.8,45.6
  Bottom 0.2: 16.8,46.2 16.8,48.3 16.2,48.9 13.2,48.9 U$4.1 | 16.8,46.2 23.1,46.2 D3.A | v16.8,45.6 16.8,46.2 | v12.6,41.4 10.8,39.6 L1.2
N$15
  Bottom 0.2: C13.1 12.9,27.9 15.9,30.9 24.6,30.9 25.8,32.1 R16.2 26.1,32.1 28.8,32.1 29.1,31.8 R17.1
N$16  (via drill 0.45)
  Top 0.2: v13.8,65.4 18.3,70.5 22.7,70.5 22.7,63.8 v20.7,62.4
  Bottom 0.2: v13.8,65.4 12,65.4 R12.1 | v20.7,62.4 20.4,62.1 19.8,62.1 U$1.1
N$17
  Bottom 0.2: R12.2 8.7,65.4 5.7,65.4 JP1.2
N$18
  Bottom 0.2: U$4.4 10.2,47.1 6,47.1 R13.1
N$19
  Bottom 0.2: R7.2 8.7,68.1 5.7,68.1 JP1.1
N$20  (via drill 0.45)
  Top 0.2: v29.4,36 31.2,37.8 31.2,41.1 32.1,42 U$3.3
  Bottom 0.2: v29.4,36 29.4,34.8 R17.2
N$21
  Bottom 0.2: R15.2 25.5,55.8 22.2,55.8 C8.1 21.9,55.8 19.8,53.7 19.2,53.7 R14.1 18.9,53.4 12,53.4 12,47.7 12.3,47.4 12.6,47.4 12.9,47.1 U$4.3
N$22  (via drill 0.45)
  Top 0.2: v51.6,73.2 51.6,69.6 v52.5,68.7 52.5,62.1 v51.2,61.5
  Bottom 0.2: R19.1 51,52.8 51,58.8 51.3,58.8 U2.1 51.6,59.1 v51.2,61.5 | v52.5,68.7 54,68.7 C14.1 | v51.6,73.2 50.7,74.1 50.1,74.1 C15.2
N$23  (via drill 0.45)
  Top 0.2: v55.5,71.7 55.2,72 v55.2,73.5
  Bottom 0.2: v55.5,71.7 54.3,71.7 54,71.4 C14.2 | v55.2,73.5 55.8,74.1 56.7,74.1 R18.1
N$24
  Bottom 0.2: U2.5 47.7,64.5 47.7,67.8 C16.1 48,68.1 49.5,69.6 57.9,69.6 58.5,70.2 60,70.2 60.3,70.5 60.3,77.1 | 60.3,77.1 64.2,77.1 R22.2 | 60.3,77.1 57,77.1 R18.2
N$25  (via drill 0.45)
  Top 0.2: v54,61.2 54.3,61.5 v54.3,63.6
  Bottom 0.2: v54,61.2 54,52.8 R19.2 | v54.3,63.6 55.5,64.8 R20.1
N$26  (via drill 0.45)
  Top 0.2: v60,65.1 60.6,65.7 v60.6,68.1
  Bottom 0.2: v60,65.1 59.1,65.1 58.8,64.8 R20.2 | v60.6,68.1 60.3,68.4 59.1,68.4 R21.1
N$27  (via drill 0.45)
  Top 0.2: v48.9,57 48.9,56.4 47.7,56.4 U$6.8
  Bottom 0.2: v48.9,57 50.1,58.2 50.1,58.8 U2.2 50.1,59.1 50.1,61.8 48.3,61.8 46.8,63.3 46.8,70.2 55.2,70.2 57.6,72.6 | 57.6,72.6 57.9,72.6 58.8,71.7 R21.2 | 57.6,72.6 53.1,72.6 52.8,72.3 49.2,72.3 47.4,74.1 C15.1
N$28
  Bottom 0.2: R22.1 64.2,74.1 64.2,71.1 R23.1 64.2,70.8 63.6,70.2 63,70.2 61.5,68.7 61.5,67.2 49.5,67.2 | 49.5,67.2 49.5,64.5 49.2,64.5 U2.6 | 49.5,67.2 49.5,67.8 C16.2
N$29  (via drill 0.45)
  Top 0.2: v64.5,60 64.2,60.3 v64.2,64.8
  Bottom 0.2: R23.2 64.2,67.8 v64.2,64.8 64.2,64.5 63.9,64.5 63.3,63.9 63.3,63.3 U$5.6 | v64.5,60 64.5,57.9 U$5.2
N$30
  Bottom 0.2: 69.3,64.5 69.3,67.8 68.4,67.8 67.5,68.7 R24.1 | 69.3,64.5 C17.1 69.3,64.5 | 69.3,64.5 65.4,64.5 65.1,64.2 64.8,64.2 64.8,63.3 U$5.7
N$31  (via drill 0.45)
  Top 0.2: v52.5,71.1 v60,63.6
  Bottom 0.2: 45.9,71.1 45.9,74.4 42.9,74.4 R25.2 | 45.9,71.1 45.9,69.3 45.6,69 43.2,69 43.2,63.3 R26.1 | v60,63.6 61.5,63.6 61.8,63.3 U$5.5 | 45.9,71.1 v52.5,71.1
N$32
  Bottom 0.2: 44.4,60.3 44.4,67.5 C18.1 | 44.4,60.3 43.2,60.3 R26.2 | 45.9,58.8 47.4,58.8 U2.4 47.7,59.1 48.9,59.1 U2.3 | 45.9,58.8 45.6,58.8 45.6,53.7 R27.1 | 45.9,58.8 44.4,60.3
N$33
  Bottom 0.2: R27.2 45.6,50.7 46.5,51.6 55.5,51.6 57.6,53.7 R28.1 57.9,54 63,54 63,57.6 U$5.3
N$34
  Bottom 0.2: R29.1 68.7,57.3 68.4,57.6 66,57.6 U$5.1
N$35
  Bottom 0.2: R29.2 72,57.3 73.8,59.1 75.3,59.1 75.9,59.7 75.9,65.4 74.7,65.4 JP2.2
N$36
  Bottom 0.2: R24.2 70.5,68.7 71.1,68.1 74.4,68.1 JP2.1
N$37
  Bottom 0.2: D2.C 63.6,54 65.4,54 R30.1 65.7,54 66.9,54 69,51.9 C20.1
N$38
  Bottom 0.2: 65.7,47.7 65.4,47.7 R31.1 65.7,47.7 | 65.7,47.7 68.4,47.7 C21.1 | 65.7,47.7 65.7,51.3 R30.2
N$39  (via drill 0.45)
  Top 0.2: v48.9,43.5 47.7,42.3 U$6.3
  Bottom 0.2: v48.9,43.5 58.5,43.5 62.4,47.4 R31.2
N$40
  Bottom 0.2: R33.1 23.7,11.1 23.7,14.1 26.4,14.1 C22.1 26.4,14.4 C23.2 28.5,17.4 29.7,18.6 U3.1
N$41  (via drill 0.45)
  Top 0.2: v32.1,3.9 v26.4,9.6
  Bottom 0.2: v26.4,9.6 C22.2 | v32.1,3.9 32.4,3.6 33.3,3.6 R32.1
N$42
  Bottom 0.2: 36.3,4.8 36.3,3.6 R32.2 | 36.3,4.8 C24.1 35.1,8.7 33.9,8.7 33.9,13.5 U3.5 | 36.3,4.8 31.2,4.8 30,3.6 R36.2
N$43
  Bottom 0.2: R33.2 20.7,11.1 20.7,14.4 21.9,14.4 23.1,15.6 R34.1
N$44
  Bottom 0.2: R34.2 20.4,15.9 20.4,20.1 R35.1
N$45  (via drill 0.45)
  Top 0.2: v28.8,20.4 32.1,23.7 U$8.8
  Bottom 0.2: R35.2 23.4,20.1 26.4,20.1 C23.1 26.4,20.4 v28.8,20.4 30.9,20.4 30.9,18.9 U3.2
N$46
  Bottom 0.2: 33.3,7.5 31.2,5.4 28.8,5.4 27,3.6 R36.1 26.7,3.6 24,3.6 R37.1 | 33.3,7.5 C24.2 33.3,7.5 | 33.3,7.5 32.4,7.5 32.4,13.5 U3.6
N$47  (via drill 0.45)
  Top 0.2: v16.2,11.1 v16.2,12.9
  Bottom 0.2: R37.2 20.7,3.6 20.7,7.8 18.3,7.8 17.7,8.4 17.7,9.3 U$7.2 17.4,9.6 17.4,10.2 16.8,10.8 16.5,10.8 v16.2,11.1 | v16.2,12.9 16.2,14.4 U$7.6
N$48  (via drill 0.45)
  Top 0.2: v14.1,7.8 17.1,10.8 v17.1,16.5
  Bottom 0.2: C25.1 17.1,20.7 v17.1,16.5 17.1,14.7 17.4,14.7 U$7.7 | v14.1,7.8 12.6,7.8 12.3,7.5 R38.1
N$49  (via drill 0.45)
  Top 0.2: v19.8,22.5 13.8,16.5 v13.8,14.4
  Bottom 0.2: R39.2 11.1,14.4 v13.8,14.4 14.7,14.4 U$7.5 | v19.8,22.5 25.8,22.5 27.3,24 R40.1
N$50  (via drill 0.45)
  Top 0.2: v36.9,19.5 36.9,20.7 36.9,22 38.6,22 arc90 38.9,22.3 38.9,22.6 38.9,25.6 38.5,26 v38.4,26.1
  Bottom 0.2: R40.2 30.6,24.3 33.9,24.3 R41.1 34.2,24 36.5,24 v38.4,26.1 | 36,18.6 C26.1 36,18.6 | 36,18.6 33.9,18.6 U3.4 33.6,18.9 32.4,18.9 U3.3 | 36,18.6 v36.9,19.5
N$51  (via drill 0.45)
  Top 0.2: v12.3,18.3 v19.5,25.5
  Bottom 0.2: U$7.3 15.9,9.6 15.9,10.2 15.3,10.8 14.4,10.8 13.8,10.2 9,10.2 9,15.6 10.8,17.4 R42.1 10.8,17.7 11.7,17.7 v12.3,18.3 | v19.5,25.5 32.7,25.5 33.9,26.7 R41.2
N$52
  Bottom 0.2: R43.1 17.7,3.6 18.9,2.4 21.9,2.4 22.2,2.7 22.2,9 19.2,9 18.9,9.3 U$7.1
N$53
  Bottom 0.2: R43.2 14.7,3.6 12.3,6 8.7,6 4.2,10.5 4.2,14.4 5.4,14.4 JP3.2
N$54
  Bottom 0.2: R38.2 9.3,7.5 5.7,11.1 5.7,12 JP3.1
N$55
  Bottom 0.2: 17.7,32.1 15.9,33.9 9,33.9 8.7,33.6 8.7,24.6 15,24.6 C28.1 | 17.7,32.1 D4.C 17.7,32.1 | 17.7,32.1 20.1,34.5 25.8,34.5 27.3,33 39.9,33 39.9,30.3 38.4,28.8 R44.1
N$56
  Bottom 0.2: C29.1 22.8,28.2 25.2,30.6 33.3,30.6 33.9,31.2 R45.1 34.2,31.5 38.1,31.5 R44.2
N$57  (via drill 0.45)
  Top 0.2: v33.9,36.3 32.4,37.8 U$8.3
  Bottom 0.2: v33.9,36.3 33.9,34.5 R45.2
N$58  (via drill 0.45)
  Top 0.2: v53.4,25.8 53.7,25.5 v53.7,19.5
  Bottom 0.2: C30.1 50.4,27.3 53.4,27.3 C31.2 53.4,27 v53.4,25.8 | 49.8,21 49.8,18.3 50.4,17.7 54.6,17.7 54.6,13.2 54.9,12.9 57.3,12.9 59.1,11.1 R47.1 | 49.8,21 48.6,21 48,20.4 48,19.8 U4.1 | v53.7,19.5 52.2,21 49.8,21
N$59
  Bottom 0.2: C30.2 47.4,27.6 47.4,30.9 47.1,30.9 R46.1
N$60  (via drill 0.45)
  Top 0.2: v44.1,27 46.8,24.3 46.8,18.6 49.2,16.2 v50.4,16.2
  Bottom 0.2: R50.2 54.9,4.2 55.2,4.2 C32.1 51.9,11.7 51.9,14.1 U4.5 51.6,14.4 51.6,15 v50.4,16.2 | v44.1,27 44.1,30.9 R46.2
N$61  (via drill 0.45)
  Top 0.2: v59.4,16.2 60.3,17.1 v60.3,25.5
  Bottom 0.2: v59.4,16.2 59.4,13.8 R47.2 | v60.3,25.5 59.7,26.1 58.8,26.1 R48.1
N$62
  Bottom 0.2: R48.2 58.8,29.4 58.8,32.4 59.4,32.4 60.6,33.6 R49.1
N$63  (via drill 0.45)
  Top 0.2: U$10.8 48,23.7 v48.9,23.7 v48.9,17.7
  Bottom 0.2: R49.2 57.9,33.6 57.6,33.6 57.6,28.8 53.4,24.6 C31.1 53.4,24.3 49.5,24.3 v48.9,23.7 | v48.9,17.7 48.9,19.5 U4.2
N$64
  Bottom 0.2: 52.2,4.2 52.2,8.4 | 52.2,4.2 51.9,4.2 R50.1 52.2,4.2 | 52.2,8.4 C32.2 52.2,8.4 | 52.2,4.2 53.7,2.7 60.6,2.7 61.8,3.9 R51.1 | 52.2,8.4 50.7,8.4 50.7,14.1 U4.6
N$65  (via drill 0.45)
  Top 0.2: v62.7,20.4 64.5,18.6 v64.5,15.3
  Bottom 0.2: R51.2 64.5,4.2 v64.5,15.3 64.5,17.1 64.2,17.1 U$9.2 | v62.7,20.4 62.7,22.2 U$9.6
N$66
  Bottom 0.2: 71.7,21 71.7,20.4 64.5,20.4 63.9,21 63.9,22.2 U$9.7 | 71.7,21 71.7,28.5 C33.1 | 71.7,21 75.6,21 75.6,13.8 75,13.2 69.9,13.2 67.8,11.1 R52.1
N$67
  Bottom 0.2: 66.9,31.5 69.9,31.5 71.4,33 R54.1 | 66.9,31.5 66.3,31.5 63,28.2 R53.2 | 66.9,31.5 66.9,22.2 65.7,21 64.5,21 64.5,23.7 64.2,24 61.5,24 61.5,22.5 U$9.5
N$68  (via drill 0.45)
  Top 0.2: v65.7,32.1 57.3,23.7 v57.3,18
  Bottom 0.2: R55.1 68.4,37.8 68.4,33.3 R54.2 68.4,33 67.5,32.1 v65.7,32.1 | 55.8,17.1 54.6,18.3 53.1,18.3 51.9,19.5 U4.4 51.6,19.5 50.7,19.5 U4.3 | 55.8,17.1 C34.1 55.8,17.1 | v57.3,18 56.4,17.1 55.8,17.1
N$69
  Bottom 0.2: R56.1 54.6,33.9 58.5,37.8 65.4,37.8 R55.2 65.7,38.1 66.9,39.3 76.2,39.3 76.2,11.4 67.5,2.7 63.6,2.7 63.6,4.5 62.7,5.4 62.7,17.1 U$9.3
N$70
  Bottom 0.2: R57.1 67.2,15.3 65.4,17.1 U$9.1
N$71
  Bottom 0.2: R57.2 70.5,15 70.8,14.7 74.4,14.7 JP4.2
N$72
  Bottom 0.2: JP4.1 71.7,12 70.8,11.1 R52.2
N$73
  Bottom 0.2: D5.C 41.1,18.9 41.4,18.9 R58.1 41.7,18.6 42.3,18.6 42.3,14.7 C36.1 | D5.C 39,21 D5.C
N$74  (via drill 0.45)
  Top 0.2: v43.8,7.5 v43.8,17.1 v43.8,22.5
  Bottom 0.2: v43.8,7.5 43.8,3.9 C37.1 | v43.8,17.1 43.8,18.6 44.4,18.6 R58.2 | v43.8,22.5 42.3,24 R59.1
N$75  (via drill 0.45)
  Top 0.2: v42.3,32.4 47.7,37.8 U$10.3
  Bottom 0.2: v42.3,32.4 42.3,27.3 R59.2

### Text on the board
tPlace: SIG | SIG | NOISE | NOISE | GND | GND | VCC | VCC | VCC | VCC | GND | GND | NOISE | NOISE | SIG | SIG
